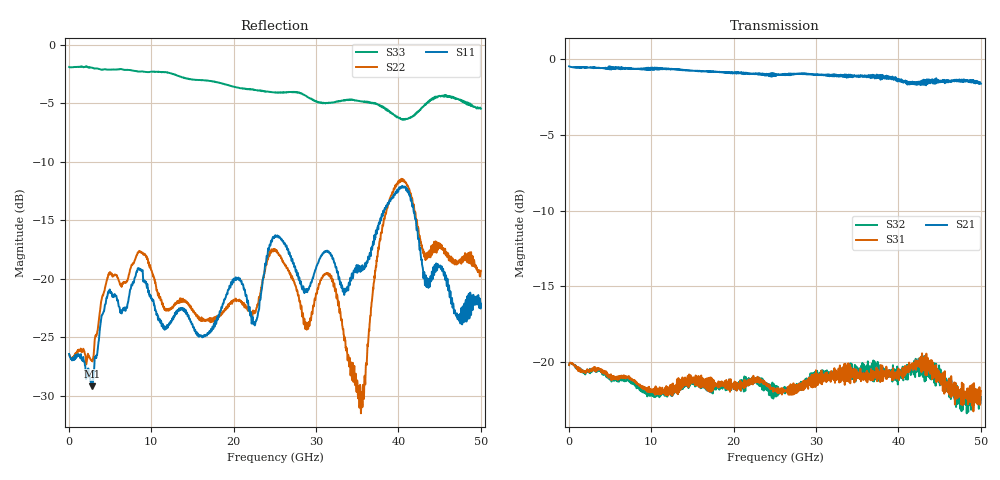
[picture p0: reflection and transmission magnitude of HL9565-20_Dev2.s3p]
! 10/7/2020 1:07:14 PM
! H:\PRODUCTION_DATA\TEMP_S3P.S3P
! CHANNEL.1
! TR.MEASUREMENT
! CORRECTED.DATA
# GHZ S RI R 50.0
! FREQ.GHZ  S11RE  S11IM  S12RE  S12IM  S13RE  S13IM
!  S21RE  S21IM  S22RE  S22IM  S23RE  S23IM
!  S31RE  S31IM  S32RE  S32IM  S33RE  S33IM
!; PortSelection: Port_123
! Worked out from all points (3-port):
!   1429 points, 35 MHz to 50.02 GHz, reference 50 ohm
!   strongest paths, dB at 35 MHz, 12.53 GHz, 25.02 GHz, 37.52 GHz, 50.02 GHz:
!     S21: -0.5, -0.7, -1.0, -1.2, -1.6
!     S31: -20.2, -21.9, -21.8, -20.5, -21.9
!     S32: -20.2, -22.0, -21.9, -20.7, -22.3
!   lowest |S11| = -29.2 dB at 2.87 GHz (marker M1), VSWR 1.07, Z = 49.7 + j3.45 ohm
!   |S11| at or under -10 dB: start of sweep to end of sweep
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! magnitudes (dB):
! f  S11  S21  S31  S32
! 35 MHz  -26.4  -0.5  -20.2  -20.2
! 2.87 GHz  -29.2  -0.5  -20.5  -20.5
! 8.54 GHz  -19.1  -0.6  -21.6  -21.8
! 16.38 GHz  -25.0  -0.8  -21.2  -21.2
! 25.02 GHz  -16.4  -1.0  -21.8  -21.9
! 28.88 GHz  -21.1  -1.0  -21.6  -21.4
! 31.82 GHz  -18.0  -1.1  -21.0  -20.9
! 35.42 GHz  -19.2  -1.0  -21.0  -20.9
! 40.01 GHz  -12.4  -1.4  -20.4  -20.5
! 50.02 GHz  -22.1  -1.6  -21.9  -22.3
